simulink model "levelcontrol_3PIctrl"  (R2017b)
settings: Solver=ode3  StartTime=0.0  StopTime=10.0  FixedStep=0.1  RelTol=1e-3
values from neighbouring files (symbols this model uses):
  d1amplitude = 0.05    [ExamplePIbased.m]    (also in levelcontrol_init3.m; levelcontrol_init4.m; levelcontrol_init5.m; levelcontrol_init6.m)
  d1bias = 0    [ExamplePIbased.m]    (also in levelcontrol_init3.m; levelcontrol_init4.m; levelcontrol_init5.m; levelcontrol_init6.m)
  d1freq = 1    [ExamplePIbased.m]    (also in levelcontrol_init3.m; levelcontrol_init4.m; levelcontrol_init5.m; levelcontrol_init6.m)
  d1phase = 0    [ExamplePIbased.m]    (also in levelcontrol_init3.m; levelcontrol_init4.m; levelcontrol_init5.m; levelcontrol_init6.m)
  d2 = 0.4    [ExamplePIbased.m]    (also in levelcontrol_init3.m = 0.2; levelcontrol_init4.m = 0.2; levelcontrol_init5.m; levelcontrol_init6.m = 0.2)
  d3 = -0.8    [ExamplePIbased.m]    (also in levelcontrol_init3.m = 0.2; levelcontrol_init4.m = 0.2; levelcontrol_init5.m; levelcontrol_init6.m = 0.2)
  d4 = 0.05    [ExamplePIbased.m]    (also in levelcontrol_init3.m = 0.1; levelcontrol_init4.m; levelcontrol_init5.m; levelcontrol_init6.m)
  d5 = -0.9    [ExamplePIbased.m]    (also in levelcontrol_init3.m; levelcontrol_init4.m; levelcontrol_init5.m; levelcontrol_init6.m)
  h0 = 0.5    [ExamplePIbased.m]    (also in levelcontrol_init3.m; levelcontrol_init4.m; levelcontrol_init5.m; levelcontrol_init6.m)
  h_set = 0.5    [ExamplePIbased.m]    (also in levelcontrol_init3.m; levelcontrol_init4.m; levelcontrol_init5.m; levelcontrol_init6.m)
  Kc = (1/kprime)*(1/(tau_c+theta))    (= -0.333333333333)    [ExamplePIbased.m]    (also in levelcontrol_init3.m; levelcontrol_init4.m; levelcontrol_init5.m; levelcontrol_init6.m)
  Kcmax = Kcmin    (= -6.66666666667)    [ExamplePIbased.m]    (also in levelcontrol_init3.m = -10; levelcontrol_init4.m; levelcontrol_init5.m; levelcontrol_init6.m)
  Kcmin = f*Kc    (= -6.66666666667)    [ExamplePIbased.m]    (also in levelcontrol_init3.m = -10; levelcontrol_init4.m; levelcontrol_init5.m; levelcontrol_init6.m)
  noise_ON = 0    [ExamplePIbased.m]    (also in levelcontrol_init3.m = 1; levelcontrol_init4.m; levelcontrol_init5.m; levelcontrol_init6.m = 1)
  p = 1    [ExamplePIbased.m]    (also in levelcontrol_init3.m; levelcontrol_init4.m; levelcontrol_init5.m; levelcontrol_init6.m)
  qin0 = 0.5    [ExamplePIbased.m]    (also in levelcontrol_init3.m; levelcontrol_init4.m; levelcontrol_init5.m; levelcontrol_init6.m)
  qout0 = 0.5    [ExamplePIbased.m]    (also in levelcontrol_init3.m; levelcontrol_init4.m; levelcontrol_init5.m; levelcontrol_init6.m)
  sin_ON = 1    [ExamplePIbased.m]    (also in levelcontrol_init3.m; levelcontrol_init4.m = 0; levelcontrol_init5.m; levelcontrol_init6.m)
  tauI = 4*(tau_c+theta)    (= 12)    [ExamplePIbased.m]    (also in levelcontrol_init3.m; levelcontrol_init4.m; levelcontrol_init5.m; levelcontrol_init6.m)
  td2 = 30    [ExamplePIbased.m]    (also in levelcontrol_init3.m = 50; levelcontrol_init4.m = 50; levelcontrol_init5.m; levelcontrol_init6.m = 50)
  td3 = 200    [ExamplePIbased.m]    (also in levelcontrol_init3.m = 100; levelcontrol_init4.m = 100; levelcontrol_init5.m; levelcontrol_init6.m = 100)
  td4 = 350    [ExamplePIbased.m]    (also in levelcontrol_init3.m = 150; levelcontrol_init4.m = 150; levelcontrol_init5.m; levelcontrol_init6.m = 150)
  td5 = 300    [ExamplePIbased.m]    (also in levelcontrol_init3.m = 200; levelcontrol_init4.m = 205; levelcontrol_init5.m; levelcontrol_init6.m = 205)
  Umaxsat = Umax-qout0    (= 0.5)    [ExamplePIbased.m]    (also in levelcontrol_init3.m; levelcontrol_init4.m; levelcontrol_init5.m; levelcontrol_init6.m)
  Uminsat = Umin-qout0    (= -0.5)    [ExamplePIbased.m]    (also in levelcontrol_init3.m; levelcontrol_init4.m; levelcontrol_init5.m; levelcontrol_init6.m)
  Ymax = 0.9-offset    (= 0.84)    [ExamplePIbased.m]    (also in levelcontrol_init3.m = 0.9; levelcontrol_init4.m; levelcontrol_init5.m; levelcontrol_init6.m)
  Ymin = 0.1+offset    (= 0.16)    [ExamplePIbased.m]    (also in levelcontrol_init3.m = 0.1; levelcontrol_init4.m; levelcontrol_init5.m; levelcontrol_init6.m)
undefined symbols (not defined in the file or in its folder): SimpleTank_ODE, tauImax, tauImin
libraries: simulink x5

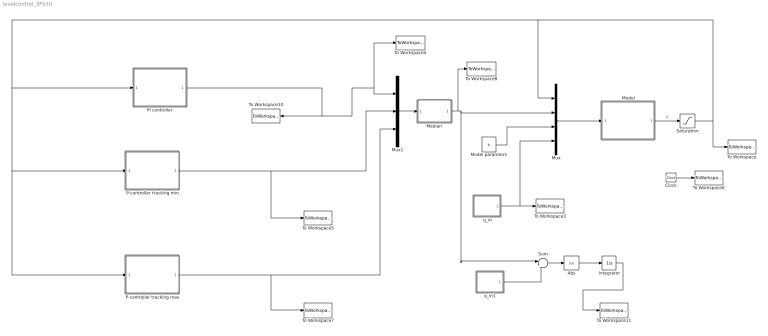
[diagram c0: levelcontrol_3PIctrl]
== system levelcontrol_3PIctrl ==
  Abs : Abs
  Clock : Clock
  Integrator : Integrator
  Median : MATLAB Function  TreatAsAtomicUnit=on
  Model : Subsystem
  Model paramters : Constant  Value=p
  Mux : Mux
  Mux1 : Mux  Inputs=3
  P-controller tracking max : Subsystem
  P-controller tracking min : Subsystem
  PI controller : Subsystem
  Saturation : Saturate  UpperLimit=1  LowerLimit=0
  Sum : Sum  Inputs=|+-
  To Workspace : ToWorkspace  VariableName=h  SaveFormat=Structure With Time  SampleTime=-1
  To Workspace10 : ToWorkspace  VariableName=q_outPI  SaveFormat=Structure With Time  SampleTime=-1
  To Workspace11 : ToWorkspace  VariableName=IAE_q  SaveFormat=Structure With Time  SampleTime=-1
  To Workspace3 : ToWorkspace  VariableName=q_in  SaveFormat=Structure With Time  SampleTime=-1
  To Workspace4 : ToWorkspace  VariableName=q_outmid  SaveFormat=Structure With Time  SampleTime=-1
  To Workspace5 : ToWorkspace  VariableName=q_outmin  SaveFormat=Structure With Time  SampleTime=-1
  To Workspace6 : ToWorkspace  VariableName=time  SampleTime=-1
  To Workspace7 : ToWorkspace  VariableName=q_outmax  SaveFormat=Structure With Time  SampleTime=-1
  To Workspace8 : ToWorkspace  VariableName=q_out  SaveFormat=Structure With Time  SampleTime=-1
  q_in : Subsystem
  q_in1 : Subsystem
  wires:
  q_in/1(q_in) -> Mux/4, To Workspace3/1
  Mux/1 -> Model/1(x,u,p,d)
  Model paramters/1 -> Mux/3
  Mux1/1 -> Median/1(u)
  Clock/1 -> To Workspace6/1
  Model/1(h) -> Saturation/1  "h"
  PI controller/1(u_mid) -> To Workspace4/1, Mux1/1, To Workspace10/1
  P-controller tracking min/1(u_min) -> To Workspace5/1, Mux1/2
  P-controller tracking max/1(u_max) -> To Workspace7/1, Mux1/3
  Median/1(y) -> Sum/1, Mux/2, To Workspace8/1
  Saturation/1 -> To Workspace/1, Mux/1, P-controller tracking max/1(h), P-controller tracking min/1(h), PI controller/1(h)
  q_in1/1(q_in) -> Sum/2
  Sum/1 -> Abs/1
  Integrator/1 -> To Workspace11/1
  Abs/1 -> Integrator/1

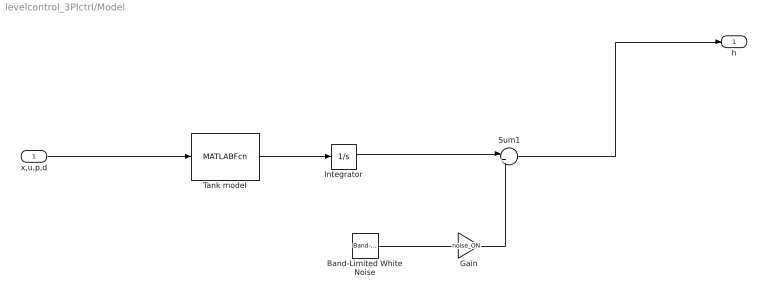
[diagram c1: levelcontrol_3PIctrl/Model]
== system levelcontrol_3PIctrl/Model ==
  x,u,p,d : Inport
  Band-Limited White Noise : simulink/Sources/Band-Limited White Noise  Cov=noise_power  Ts=0.1  seed=[23341]
  Gain : Gain  Gain=noise_ON
  Integrator : Integrator  InitialCondition=h0
  Sum1 : Sum  Inputs=|++
  Tank model : MATLABFcn  MATLABFcn=SimpleTank_ODE(u(1),u(2),u(3),u(4))  OutputDimensions=1
  h : Outport
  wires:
  Tank model/1 -> Integrator/1
  Sum1/1 -> h/1
  x,u,p,d/1 -> Tank model/1
  Integrator/1 -> Sum1/1
  Band-Limited White Noise/1 -> Gain/1
  Gain/1 -> Sum1/2

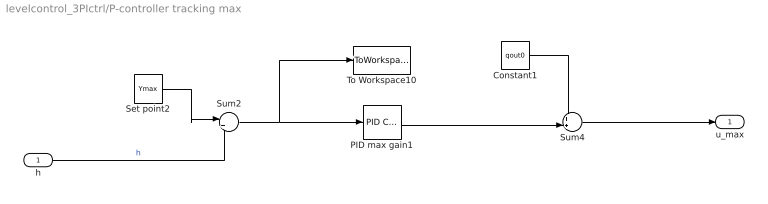
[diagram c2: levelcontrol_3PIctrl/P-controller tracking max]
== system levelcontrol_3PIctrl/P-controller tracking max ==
  h : Inport
  Constant1 : Constant  Value=qout0
  PID max gain1 : simulink/Continuous/PID Controller  Controller=P  TimeDomain=Continuous-time  SampleTime=-1  IntegratorMethod=Forward Euler  FilterMethod=Forward Euler  Form=Parallel  UseFilter=on  ControllerParametersSource=internal  P=Kcmax  I=Kcmax/tauImax  D=0  N=100  InitialConditionSource=internal  InitialConditionForIntegrator=0  InitialConditionForFilter=0  ExternalReset=none  LimitOutput=on  UpperSaturationLimit=Umaxsat  LowerSaturationLimit=Uminsat  LinearizeAsGain=on  AntiWindupMode=back-calculation  Kb=1  TrackingMode=on  Kt=1  PParamMin=[]  PParamMax=[]  IParamMin=[]  IParamMax=[]  DParamMin=[]  DParamMax=[]  NParamMin=[]  NParamMax=[]  KbParamMin=[]  KbParamMax=[]  KtParamMin=[]  KtParamMax=[]  POutMin=[]  POutMax=[]  IOutMin=[]  IOutMax=[]  DOutMin=[]  DOutMax=[]  NOutMin=[]  NOutMax=[]  KbOutMin=[]  KbOutMax=[]  KtOutMin=[]  KtOutMax=[]  IntegratorOutMin=[]  IntegratorOutMax=[]  FilterOutMin=[]  FilterOutMax=[]  SumOutMin=[]  SumOutMax=[]  SumI1OutMin=[]  SumI1OutMax=[]  SumI2OutMin=[]  SumI2OutMax=[]  SumI3OutMin=[]  SumI3OutMax=[]  SumDOutMin=[]  SumDOutMax=[]  SaturationOutMin=[]  SaturationOutMax=[]  IntegratorContinuousStateAttributes=''  IntegratorStateMustResolveToSignalObject=off  IntegratorRTWStateStorageClass=Auto  FilterContinuousStateAttributes=''  FilterStateMustResolveToSignalObject=off  FilterRTWStateStorageClass=Auto  DifferentiatorICPrevScaledInput=0  DifferentiatorOutMin=[]  DifferentiatorOutMax=[]  InitialConditionSetting=State (most efficient)  FilterDiffOutCoefMin=[]  FilterDiffOutCoefMax=[]  SumDenOutMin=[]  SumDenOutMax=[]  SumNumOutMin=[]  SumNumOutMax=[]  ReciprocalOutMin=[]  ReciprocalOutMax=[]  DivideOutMin=[]  DivideOutMax=[]  TunerSelectOption=Transfer Function Based (PID Tuner App)
  Set point2 : Constant  Value=Ymax
  Sum2 : Sum  Inputs=|+-
  Sum4 : Sum  Inputs=++|
  To Workspace10 : ToWorkspace  VariableName=emax  SampleTime=-1
  u_max : Outport
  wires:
  Set point2/1 -> Sum2/1
  h/1 -> Sum2/2  "h"
  Sum2/1 -> PID max gain1/1, To Workspace10/1
  Sum4/1 -> u_max/1
  Constant1/1 -> Sum4/1
  PID max gain1/1 -> Sum4/2

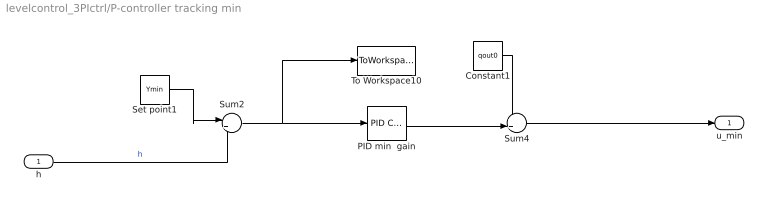
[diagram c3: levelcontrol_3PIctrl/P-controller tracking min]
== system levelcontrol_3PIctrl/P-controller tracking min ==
  h : Inport
  Constant1 : Constant  Value=qout0
  PID min  gain : simulink/Continuous/PID Controller  Controller=P  TimeDomain=Continuous-time  SampleTime=-1  IntegratorMethod=Forward Euler  FilterMethod=Forward Euler  Form=Parallel  UseFilter=on  ControllerParametersSource=internal  P=Kcmin  I=Kcmin/tauImin  D=0  N=100  InitialConditionSource=internal  InitialConditionForIntegrator=0  InitialConditionForFilter=0  ExternalReset=none  LimitOutput=on  UpperSaturationLimit=Umaxsat  LowerSaturationLimit=Uminsat  LinearizeAsGain=on  AntiWindupMode=back-calculation  Kb=1  TrackingMode=on  Kt=1  PParamMin=[]  PParamMax=[]  IParamMin=[]  IParamMax=[]  DParamMin=[]  DParamMax=[]  NParamMin=[]  NParamMax=[]  KbParamMin=[]  KbParamMax=[]  KtParamMin=[]  KtParamMax=[]  POutMin=[]  POutMax=[]  IOutMin=[]  IOutMax=[]  DOutMin=[]  DOutMax=[]  NOutMin=[]  NOutMax=[]  KbOutMin=[]  KbOutMax=[]  KtOutMin=[]  KtOutMax=[]  IntegratorOutMin=[]  IntegratorOutMax=[]  FilterOutMin=[]  FilterOutMax=[]  SumOutMin=[]  SumOutMax=[]  SumI1OutMin=[]  SumI1OutMax=[]  SumI2OutMin=[]  SumI2OutMax=[]  SumI3OutMin=[]  SumI3OutMax=[]  SumDOutMin=[]  SumDOutMax=[]  SaturationOutMin=[]  SaturationOutMax=[]  IntegratorContinuousStateAttributes=''  IntegratorStateMustResolveToSignalObject=off  IntegratorRTWStateStorageClass=Auto  FilterContinuousStateAttributes=''  FilterStateMustResolveToSignalObject=off  FilterRTWStateStorageClass=Auto  DifferentiatorICPrevScaledInput=0  DifferentiatorOutMin=[]  DifferentiatorOutMax=[]  InitialConditionSetting=State (most efficient)  FilterDiffOutCoefMin=[]  FilterDiffOutCoefMax=[]  SumDenOutMin=[]  SumDenOutMax=[]  SumNumOutMin=[]  SumNumOutMax=[]  ReciprocalOutMin=[]  ReciprocalOutMax=[]  DivideOutMin=[]  DivideOutMax=[]  TunerSelectOption=Transfer Function Based (PID Tuner App)
  Set point1 : Constant  Value=Ymin
  Sum2 : Sum  Inputs=|+-
  Sum4 : Sum  Inputs=++|
  To Workspace10 : ToWorkspace  VariableName=emin1  SampleTime=-1
  u_min : Outport
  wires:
  Set point1/1 -> Sum2/1
  h/1 -> Sum2/2  "h"
  Sum2/1 -> To Workspace10/1, PID min  gain/1
  Constant1/1 -> Sum4/1
  PID min  gain/1 -> Sum4/2
  Sum4/1 -> u_min/1

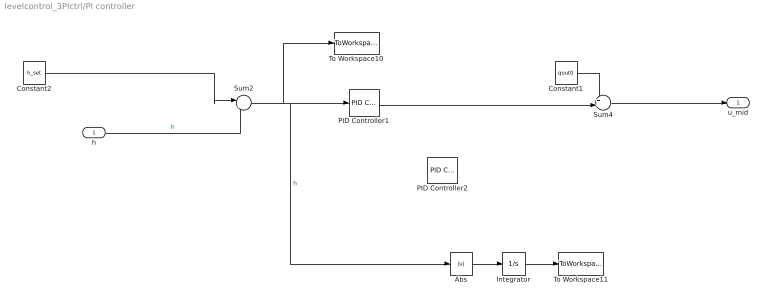
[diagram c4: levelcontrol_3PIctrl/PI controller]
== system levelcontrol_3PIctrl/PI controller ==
  h : Inport
  Abs : Abs
  Constant1 : Constant  Value=qout0
  Constant2 : Constant  Value=h_set
  Integrator : Integrator
  PID Controller1 : simulink/Continuous/PID Controller  Controller=PI  TimeDomain=Continuous-time  SampleTime=-1  IntegratorMethod=Forward Euler  FilterMethod=Forward Euler  Form=Parallel  UseFilter=on  ControllerParametersSource=internal  P=Kc  I=Kc/tauI  D=0  N=100  InitialConditionSource=internal  InitialConditionForIntegrator=0  InitialConditionForFilter=0  ExternalReset=none  LimitOutput=on  UpperSaturationLimit=Umaxsat  LowerSaturationLimit=Uminsat  LinearizeAsGain=on  AntiWindupMode=none  Kb=1  TrackingMode=off  Kt=1  PParamMin=[]  PParamMax=[]  IParamMin=[]  IParamMax=[]  DParamMin=[]  DParamMax=[]  NParamMin=[]  NParamMax=[]  KbParamMin=[]  KbParamMax=[]  KtParamMin=[]  KtParamMax=[]  POutMin=[]  POutMax=[]  IOutMin=[]  IOutMax=[]  DOutMin=[]  DOutMax=[]  NOutMin=[]  NOutMax=[]  KbOutMin=[]  KbOutMax=[]  KtOutMin=[]  KtOutMax=[]  IntegratorOutMin=[]  IntegratorOutMax=[]  FilterOutMin=[]  FilterOutMax=[]  SumOutMin=[]  SumOutMax=[]  SumI1OutMin=[]  SumI1OutMax=[]  SumI2OutMin=[]  SumI2OutMax=[]  SumI3OutMin=[]  SumI3OutMax=[]  SumDOutMin=[]  SumDOutMax=[]  SaturationOutMin=[]  SaturationOutMax=[]  IntegratorContinuousStateAttributes=''  IntegratorStateMustResolveToSignalObject=off  IntegratorRTWStateStorageClass=Auto  FilterContinuousStateAttributes=''  FilterStateMustResolveToSignalObject=off  FilterRTWStateStorageClass=Auto  DifferentiatorICPrevScaledInput=0  DifferentiatorOutMin=[]  DifferentiatorOutMax=[]  InitialConditionSetting=State (most efficient)  FilterDiffOutCoefMin=[]  FilterDiffOutCoefMax=[]  SumDenOutMin=[]  SumDenOutMax=[]  SumNumOutMin=[]  SumNumOutMax=[]  ReciprocalOutMin=[]  ReciprocalOutMax=[]  DivideOutMin=[]  DivideOutMax=[]  TunerSelectOption=Transfer Function Based (PID Tuner App)
  PID Controller2 : simulink/Continuous/PID Controller  Controller=PI  TimeDomain=Continuous-time  SampleTime=-1  IntegratorMethod=Forward Euler  FilterMethod=Forward Euler  Form=Parallel  UseFilter=on  ControllerParametersSource=internal  P=Kc  I=Kc/tauI  D=0  N=100  InitialConditionSource=internal  InitialConditionForIntegrator=0  InitialConditionForFilter=0  ExternalReset=none  LimitOutput=on  UpperSaturationLimit=Umaxsat  LowerSaturationLimit=Uminsat  LinearizeAsGain=on  AntiWindupMode=none  Kb=1  TrackingMode=off  Kt=1  PParamMin=[]  PParamMax=[]  IParamMin=[]  IParamMax=[]  DParamMin=[]  DParamMax=[]  NParamMin=[]  NParamMax=[]  KbParamMin=[]  KbParamMax=[]  KtParamMin=[]  KtParamMax=[]  POutMin=[]  POutMax=[]  IOutMin=[]  IOutMax=[]  DOutMin=[]  DOutMax=[]  NOutMin=[]  NOutMax=[]  KbOutMin=[]  KbOutMax=[]  KtOutMin=[]  KtOutMax=[]  IntegratorOutMin=[]  IntegratorOutMax=[]  FilterOutMin=[]  FilterOutMax=[]  SumOutMin=[]  SumOutMax=[]  SumI1OutMin=[]  SumI1OutMax=[]  SumI2OutMin=[]  SumI2OutMax=[]  SumI3OutMin=[]  SumI3OutMax=[]  SumDOutMin=[]  SumDOutMax=[]  SaturationOutMin=[]  SaturationOutMax=[]  IntegratorContinuousStateAttributes=''  IntegratorStateMustResolveToSignalObject=off  IntegratorRTWStateStorageClass=Auto  FilterContinuousStateAttributes=''  FilterStateMustResolveToSignalObject=off  FilterRTWStateStorageClass=Auto  DifferentiatorICPrevScaledInput=0  DifferentiatorOutMin=[]  DifferentiatorOutMax=[]  InitialConditionSetting=State (most efficient)  FilterDiffOutCoefMin=[]  FilterDiffOutCoefMax=[]  SumDenOutMin=[]  SumDenOutMax=[]  SumNumOutMin=[]  SumNumOutMax=[]  ReciprocalOutMin=[]  ReciprocalOutMax=[]  DivideOutMin=[]  DivideOutMax=[]  TunerSelectOption=Transfer Function Based (PID Tuner App)
  Sum2 : Sum  Inputs=|+-
  Sum4 : Sum  Inputs=++|
  To Workspace10 : ToWorkspace  VariableName=emid  SampleTime=-1
  To Workspace11 : ToWorkspace  VariableName=IAEmid  SaveFormat=Structure With Time  SampleTime=-1
  u_mid : Outport
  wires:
  h/1 -> Sum2/2  "h"
  Sum4/1 -> u_mid/1
  Constant1/1 -> Sum4/1
  PID Controller1/1 -> Sum4/2
  Constant2/1 -> Sum2/1
  Abs/1 -> Integrator/1
  Sum2/1 -> Abs/1, PID Controller1/1, To Workspace10/1  "h"
  Integrator/1 -> To Workspace11/1

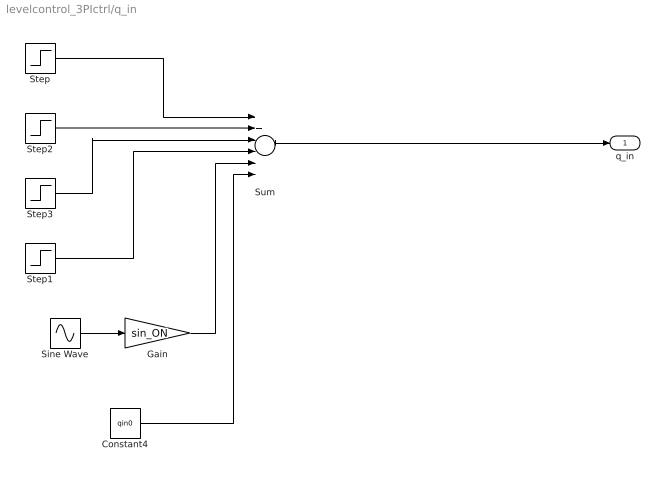
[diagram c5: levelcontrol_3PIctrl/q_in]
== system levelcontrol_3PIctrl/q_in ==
  Constant4 : Constant  Value=qin0
  Gain : Gain  Gain=sin_ON
  Sine Wave : Sin  Amplitude=d1amplitude  Bias=d1bias  Frequency=d1freq  Phase=d1phase  SampleTime=0
  Step : Step  Time=td2  After=d2  SampleTime=0
  Step1 : Step  Time=td5  After=d5  SampleTime=0
  Step2 : Step  Time=td3  After=d3  SampleTime=0
  Step3 : Step  Time=td4  After=d4  SampleTime=0
  Sum : Sum  Inputs=6
  q_in : Outport
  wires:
  Sum/1 -> q_in/1
  Step/1 -> Sum/1
  Step1/1 -> Sum/4
  Sine Wave/1 -> Gain/1
  Gain/1 -> Sum/5
  Step2/1 -> Sum/2
  Step3/1 -> Sum/3
  Constant4/1 -> Sum/6

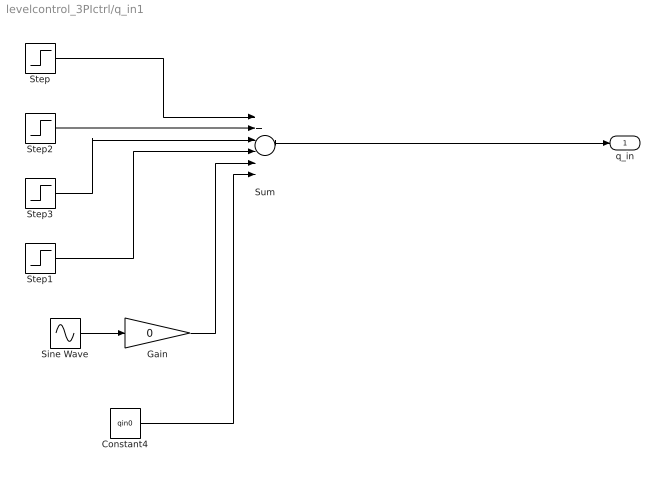
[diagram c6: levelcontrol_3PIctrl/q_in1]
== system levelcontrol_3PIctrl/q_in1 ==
  Constant4 : Constant  Value=qin0
  Gain : Gain  Gain=0
  Sine Wave : Sin  Amplitude=d1amplitude  Bias=d1bias  Frequency=d1freq  Phase=d1phase  SampleTime=0
  Step : Step  Time=td2  After=d2  SampleTime=0
  Step1 : Step  Time=td5  After=d5  SampleTime=0
  Step2 : Step  Time=td3  After=d3  SampleTime=0
  Step3 : Step  Time=td4  After=d4  SampleTime=0
  Sum : Sum  Inputs=6
  q_in : Outport
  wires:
  Sum/1 -> q_in/1
  Step/1 -> Sum/1
  Step1/1 -> Sum/4
  Sine Wave/1 -> Gain/1
  Gain/1 -> Sum/5
  Step2/1 -> Sum/2
  Step3/1 -> Sum/3
  Constant4/1 -> Sum/6

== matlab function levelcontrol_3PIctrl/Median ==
function y = fcn(u)

y = median(u);
